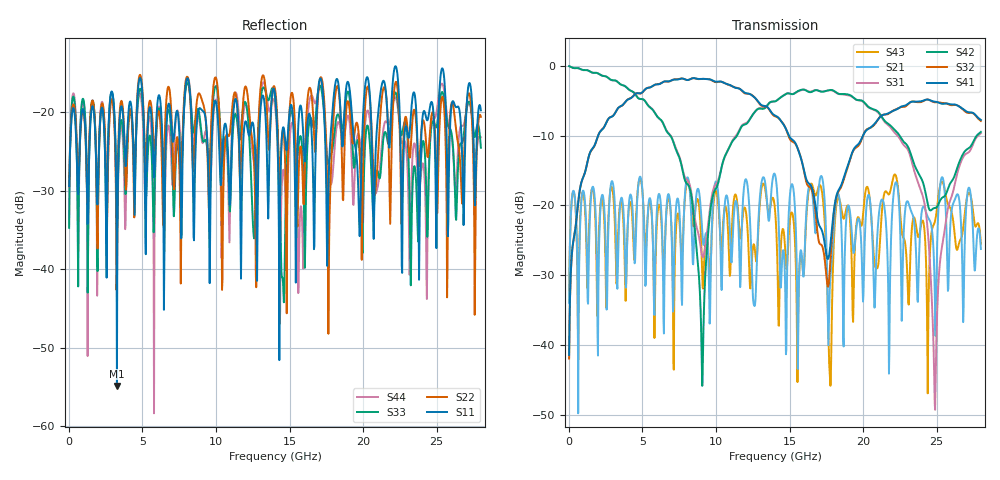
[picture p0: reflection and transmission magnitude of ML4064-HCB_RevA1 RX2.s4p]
! TOUCHSTONE file generated by CST DESIGN STUDIO
! Date and time: Wed Aug 26 10:35:09 2020
! Project name:  Project name: C:\Users\Simulation2\Temp\DE66\Untitled_0.cst
! Tree item: Tasks\SPara1\S-Parameters
# GHz S MA R 50
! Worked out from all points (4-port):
!   1000 points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, 28 MHz to 28 GHz, reference 50 ohm
!   strongest paths, dB at 28 MHz, 7.028 GHz, 14.03 GHz, 21.03 GHz, 28 GHz:
!     S41: -41.4, -2.1, -7.1, -7.6, -7.8
!     S32: -41.9, -2.1, -7.3, -7.7, -7.9
!     S42: -0.1, -10.5, -5.1, -6.6, -9.5
!     S31: -0.1, -10.4, -5.1, -6.7, -9.7
!     S21: -33.9, -27.5, -15.7, -22.3, -26.2
!     S43: -33.7, -26.2, -20.9, -28.5, -25.5
!   lowest |S11| = -54.8 dB at 3.276 GHz (marker M1), VSWR 1.00, Z = 49.9 - j0.14 ohm
!   |S11| at or under -10 dB: start of sweep to end of sweep
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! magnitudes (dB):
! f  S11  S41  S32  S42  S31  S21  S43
! 28 MHz  -29.4  -41.4  -41.9  -0.1  -0.1  -33.9  -33.7
! 3.276 GHz  -54.8  -6.3  -6.3  -2.2  -2.3  -31.1  -30.6
! 9.072 GHz  -19.8  -1.9  -1.9  -45.8  -27.2  -23.9  -30.1
! 17.58 GHz  -37.2  -27.6  -31.5  -3.6  -3.6  -33.2  -33.6
! 19.91 GHz  -24.7  -10.4  -10.5  -5.0  -5.1  -27.4  -22.8
! 24.86 GHz  -23.7  -5.2  -5.2  -20.4  -48.3  -32.2  -22.4
! 28 GHz  -19.7  -7.8  -7.9  -9.5  -9.7  -26.2  -25.5
